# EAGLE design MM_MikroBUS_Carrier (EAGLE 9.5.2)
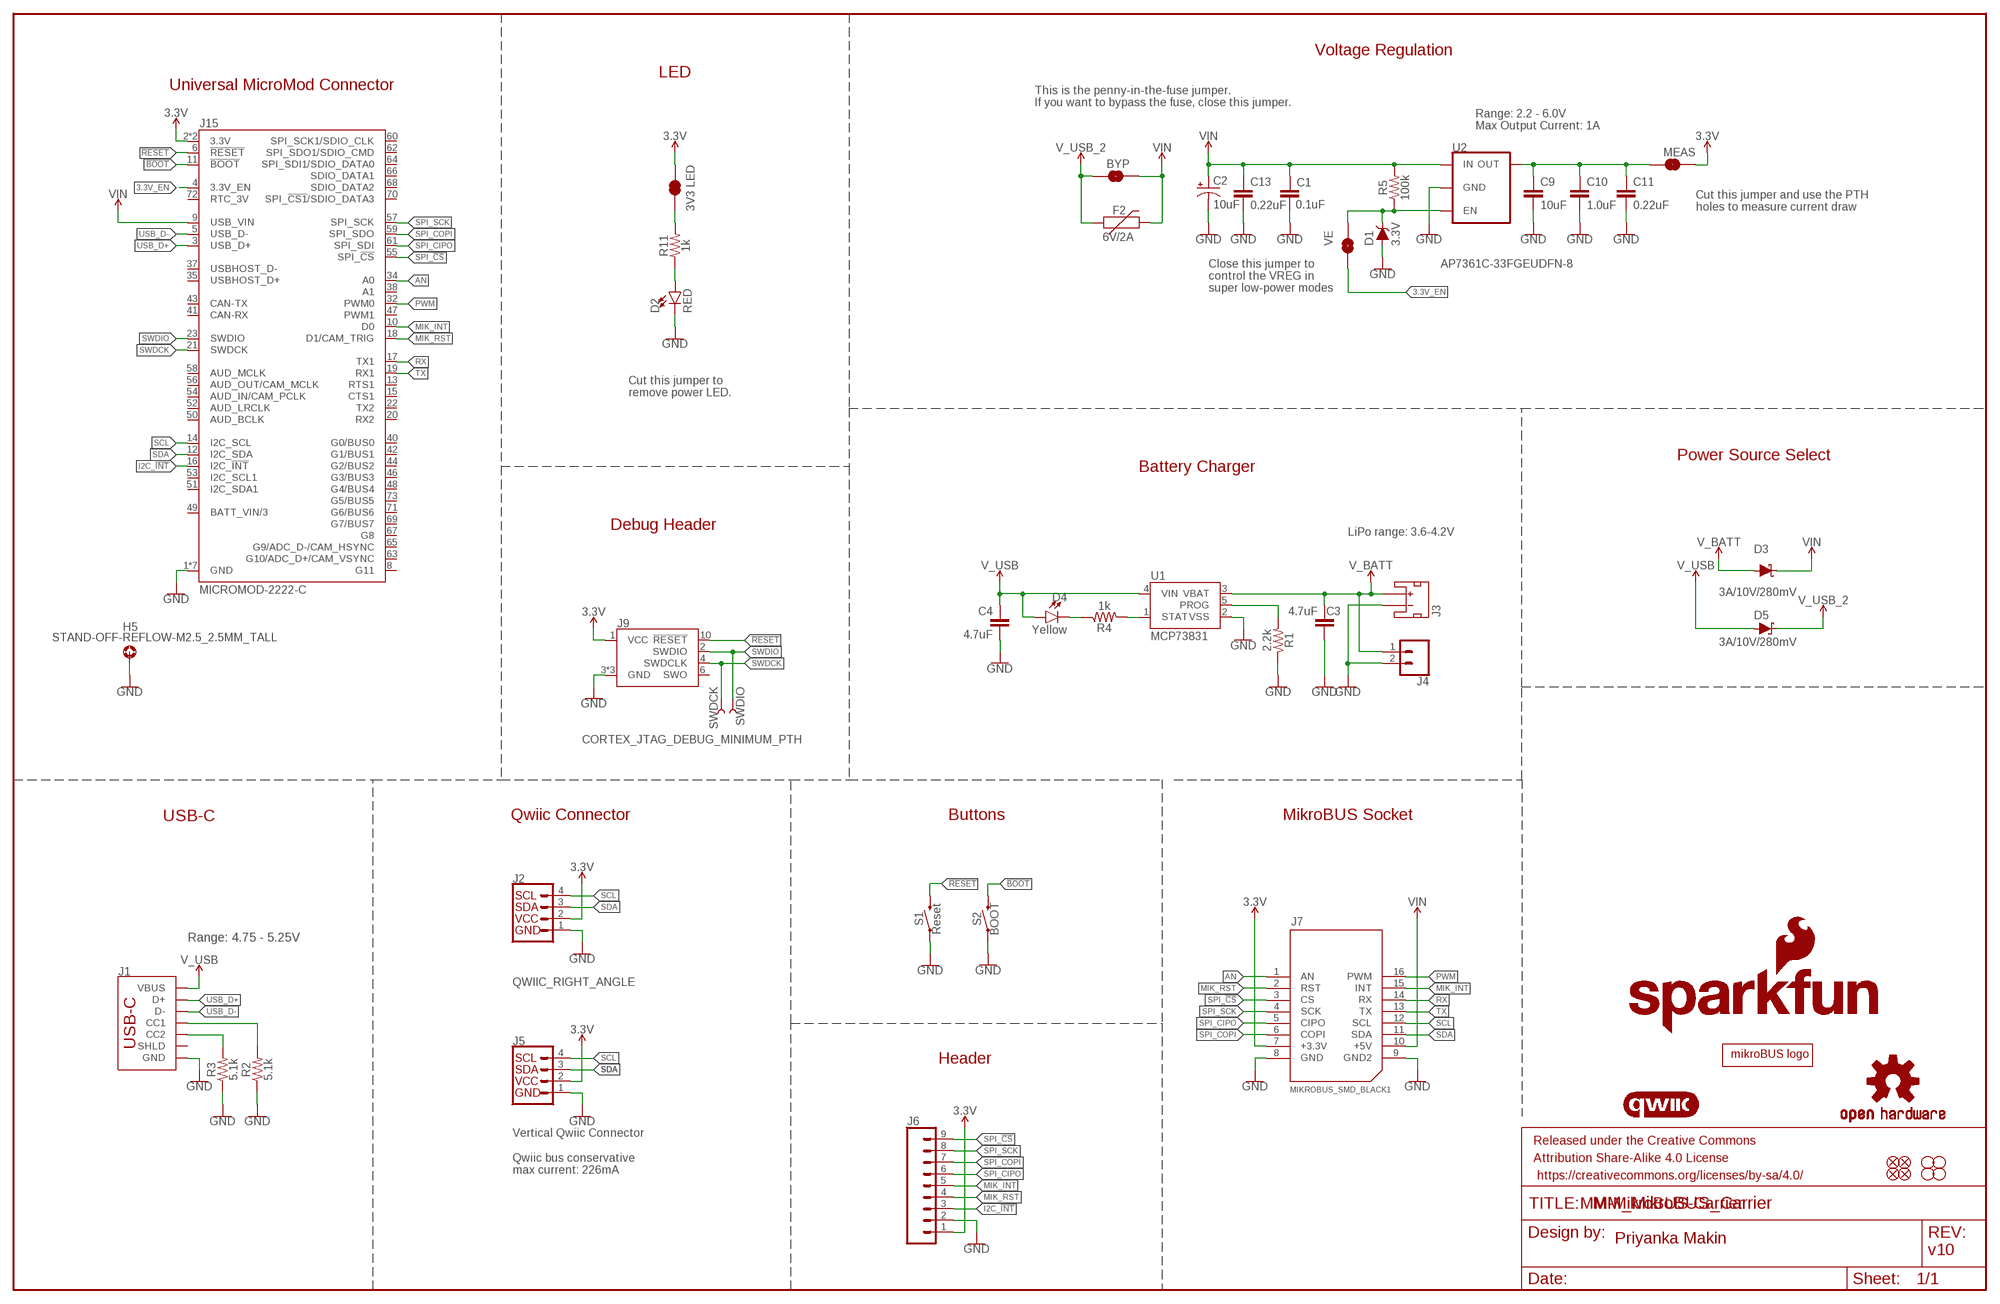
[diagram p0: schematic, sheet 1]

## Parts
BYP  JUMPER-SMT_2_NO_SILK  [SMT-JUMPER_2_NO_SILK]
C1  0.1uF  0.1UF-0603-25V-(+80/-20%)  [0603]
C2  10uF  10UF-POLAR-EIA3216-16V-10%(TANT)  [EIA3216]
C3  4.7uF  4.7UF-0603-35V-(20%)  [0603]
C4  4.7uF  4.7UF-0603-35V-(20%)  [0603]
C9  10uF  10UF-0603-6.3V-20%  [0603]
C10  1.0uF  1.0UF-0603-16V-10%  [0603]
C11  0.22uF  0.22UF-0603-25V-10%  [0603]
C13  0.22uF  0.22UF-0603-25V-10%  [0603]
D1  3.3V  DIODE-ZENER-MM3Z3V3T1G  [SOD-323]
D2  RED  LED-RED0603  [LED-0603]
D3  3A/10V/280mV  DIODE-SCHOTTKY-BAT60A  [SOD-323]
D4  Yellow  LED-YELLOW0603  [LED-0603]
D5  3A/10V/280mV  DIODE-SCHOTTKY-BAT60A  [SOD-323]
F2  6V/2A  PPTC_6V2A  [1210]
FD1  FIDUCIALUFIDUCIAL  [FIDUCIAL-MICRO]
FD2  FIDUCIALUFIDUCIAL  [FIDUCIAL-MICRO]
FD3  FIDUCIALUFIDUCIAL  [FIDUCIAL-MICRO]
FD4  FIDUCIALUFIDUCIAL  [FIDUCIAL-MICRO]
FRAME1  FRAME-LEDGER  [CREATIVE_COMMONS]
H1  STAND-OFF  [STAND-OFF]
H2  STAND-OFF  [STAND-OFF]
H3  STAND-OFF  [STAND-OFF]
H4  STAND-OFF  [STAND-OFF]
H5  STAND-OFF-REFLOW-M2.5_2.5MM_TALL  [STAND-OFF-REFLOW-M2.5]
J1  USB_C_2-LAYER_PADS  [USB-C-16P-2LAYER-PADS]
J2  QWIIC_RIGHT_ANGLE  QWIIC_CONNECTORJS-1MM  [JST04_1MM_RA]
J3  JST_2MM_MALE  [JST-2-SMD]
J4  CONN_021X02_NO_SILK  [1X02_NO_SILK]
J5  Vertical Qwiic Connector  QWIIC_CONNECTOR  [JST04_1MM_VERT]
J6  CONN_09NO_SILK  [1X09_NO_SILK]
J7  MIKROBUS_SMD_BLACK1  [MIKROBUS_SMD_BLACK]
J9  CORTEX_JTAG_DEBUG_MINIMUM_PTH  [2X5-PTH-1.27MM]
J15  MICROMOD-2222-C  [M.2-CONNECTOR-E]
JP4  3V3 LED  JUMPER-SMT_2_NC_TRACE_SILK  [SMT-JUMPER_2_NC_TRACE_SILK]
JP6  VE  JUMPER-SMT_2_NO_SILK  [SMT-JUMPER_2_NO_SILK]
LOGO1  SFE_LOGO_NAME_FLAME.2_INCH  [SFE_LOGO_NAME_FLAME_.2]
LOGO2  QWIIC_LOGO_CONNECTOR  [QWIIC_5.5MM]
LOGO3  OSHW-LOGOM  [OSHW-LOGO-M]
MEAS  JUMPER-COMBO_2_NC_TRACE  [COMBO-JUMPER_2_NC_TRACE]
R1  2.2k  2.2KOHM-0603-1/10W-1%  [0603]
R2  5.1k  5.1KOHM5.1KOHM-0603-1/10W-1%  [0603]
R3  5.1k  5.1KOHM5.1KOHM-0603-1/10W-1%  [0603]
R4  1k  1KOHM-0603-1/10W-1%  [0603]
R5  100k  100KOHM-0603-1/10W-1%  [0603]
R11  1k  1KOHM-0603-1/10W-1%  [0603]
S1  Reset  MOMENTARY-SWITCH-SPST-SMD-5.2-TALL-REDUNDANT  [TACTILE_SWITCH_SMD_5.2MM]
S2  BOOT  MOMENTARY-SWITCH-SPST-SMD-5.2-TALL-REDUNDANT  [TACTILE_SWITCH_SMD_5.2MM]
SWDCK  TEST-POINTTP_15TH_THRU  [TP_15TH]
SWDIO  TEST-POINTTP_15TH_THRU  [TP_15TH]
U1  MCP73831  [SOT23-5]
U2  AP7361C-33FGEUDFN-8  [UDFN-8]
U$7  MIKROBUS_LOGO  [MIKROBUS_LOGO]

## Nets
3.3V: J2.2 J5.2 J6.1 J7.7(+3.3V) J9.1(VCC) J15.2(3.3V) J15.74(3.3V) JP4.2 MEAS.2 MEAS.4
3.3V_EN: J15.4(3.3V_EN) JP6.1
!BOOT!: J15.11(!BOOT!) S2.3 S2.4
!RESET!: J9.10(!RESET) J15.6(!RESET!) S1.3 S1.4
AN: J7.1(AN) J15.34(A0)
GND: C1.2 C2.- C3.2 C4.2 C9.2 C10.2 C11.2 C13.2 D1.A D2.C H5.1 J1.GND J1.GND2(GND) J2.1 J3.1(-) J4.2 J5.1 J6.2 J7.8(GND) J7.9(GND2) J9.3(GND) J9.5(GND) J9.9(GND) J15.1(GND) J15.7(GND) J15.33(GND) J15.36(GND) J15.39(GND) J15.45(GND) J15.75(GND) R1.1 R2.1 R3.1 S1.1 S1.2 S2.1 S2.2 U1.2(VSS) U2.4(GND) U2.EP(GND)
I2C_!INT!: J6.3 J15.16(I2C_!INT!)
MIK_INT: J6.5 J7.15(INT) J15.10(D0)
MIK_RST: J6.4 J7.2(RST) J15.18(D1/CAM_TRIG)
N$1: C9.1 C10.1 C11.1 MEAS.1 MEAS.3 U2.1(OUT)
N$2: R1.2 U1.5(PROG)
N$3: D4.C R4.1
N$4: JP4.1 R11.2
N$6: D2.A R11.1
N$8: R4.2 U1.1(STAT)
N$10: J1.A5(CC1) R2.2
N$11: J1.B5(CC2) R3.2
PWM: J7.16(PWM) J15.32(PWM0)
RX: J7.14(RX) J15.17(TX1)
SCL: J2.4 J5.4 J7.12(SCL) J15.14(I2C_SCL)
SDA: J2.3 J5.3 J7.11(SDA) J15.12(I2C_SDA)
SPI_!CS!: J6.9 J7.3(CS) J15.55(SPI_!CS!)
SPI_CIPO: J6.6 J7.5(CIPO) J15.61(SPI_SDI)
SPI_COPI: J6.7 J7.6(COPI) J15.59(SPI_SDO)
SPI_SCK: J6.8 J7.4(SCK) J15.57(SPI_SCK)
SWDCK: J9.4(SWDCLK) J15.21(SWDCK) SWDCK.1
SWDIO: J9.2(SWDIO) J15.23(SWDIO) SWDIO.1
TX: J7.13(TX) J15.19(RX1)
USB_D+: J1.A6(D+) J1.B6(D+) J15.3(USB_D+)
USB_D-: J1.A7(D-) J1.B7(D-) J15.5(USB_D-)
V_BATT: C3.1 D3.A J3.2(+) J4.1 U1.3(VBAT)
V_USB: C4.1 D4.A D5.A J1.VBUS1(VBUS) J1.VBUS2(VBUS) U1.4(VIN)
V_USB_2: BYP.1 D5.C F2.1
VIN: BYP.2 C1.1 C2.+ C13.1 D3.C F2.2 J7.10(+5V) J15.9(USB_VIN) R5.2 U2.8(IN)
VREG_EN: D1.C JP6.2 R5.1 U2.5(EN)
Unconnected: J1.SHLD1(SHLD) J1.SHLD2(SHLD) J1.SHLD3(SHLD) J1.SHLD4(SHLD) J3.NC1(PAD1) J3.NC2(PAD2) J9.6(SWO) J15.8(G11) J15.13(RTS1) J15.15(CTS1) J15.20(RX2) J15.22(TX2) J15.35(USBHOST_D+) J15.37(USBHOST_D-) J15.38(A1) J15.40(G0/BUS0) J15.41(CAN-RX) J15.42(G1/BUS1) J15.43(CAN-TX) J15.44(G2/BUS2) J15.46(G3/BUS3) J15.47(PWM1) J15.48(G4/BUS4) J15.49(BATT_VIN/3) J15.50(AUD_BCLK) J15.51(I2C_SDA1) J15.52(AUD_LRCLK) J15.53(I2C_SCL1) J15.54(AUD_IN/CAM_PCLK) J15.56(AUD_OUT/CAM_MCLK) J15.58(AUD_MCLK) J15.60(SPI_SCK1/SDIO_CLK) J15.62(SPI_SDO1/SDIO_CMD) J15.63(G10/ADC_D+/CAM_VSYNC) J15.64(SPI_SDI1/SDIO_DATA0) J15.65(G9/ADC_D-/CAM_HSYNC) J15.66(SDIO_DATA1) J15.67(G8) J15.68(SDIO_DATA2) J15.69(G7/BUS7) J15.70(SPI_!CS1!/SDIO_DATA3) J15.71(G6/BUS6) J15.72(RTC_3V) J15.73(G5/BUS5)

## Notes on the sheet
- Voltage Regulation
- LED
- Universal MicroMod Connector
- This is the penny-in-the-fuse jumper.
  If you want to bypass the fuse, close this jumper.
- Range: 2.2 - 6.0V
  Max Output Current: 1A
- Cut this jumper and use the PTH 
  holes to measure current draw
- Close this jumper to 
  control the VREG in 
  super low-power modes
- Cut this jumper to
  remove power LED.
- Power Source Select
- Battery Charger
- Debug Header
- LiPo range: 3.6-4.2V
- USB-C | Qwiic Connector | Buttons | MikroBUS Socket
- Range: 4.75 - 5.25V
- Header
- Qwiic bus conservative 
  max current: 226mA
- MM-MikroBUS-Carrier
- Priyanka Makin
- v10

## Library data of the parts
BYP JP6 = SparkFun-Jumpers:JUMPER-SMT_2_NO: Normally open jumper
C1 = SparkFun-Capacitors:0.1UF: 0.1µF ceramic capacitors; PROD_ID: CAP-00810
C2 = SparkFun-Capacitors:10UF-POLAR: 10.0µF polarized capacitors; PROD_ID: CAP-00811
C3 C4 = SparkFun-Capacitors:4.7UF: 4.7µF ceramic capacitors; PROD_ID: CAP-14106
C9 = SparkFun-Capacitors:10UF: 10.0µF ceramic capacitors; PROD_ID: CAP-11015
C10 = SparkFun-Capacitors:1.0UF: 1µF ceramic capacitors; PROD_ID: CAP-00868
C11 C13 = SparkFun-Capacitors:0.22UF: 0.22µF ceramic capacitors; PROD_ID: CAP-07822
D1 = SparkFun-DiscreteSemi:DIODE-ZENER: Zener Diode; PROD_ID: DIO-11284
D2 = SparkFun-LED:LED-RED: Red SMD LED; PROD_ID: DIO-00819
D3 D5 = SparkFun-DiscreteSemi:DIODE-SCHOTTKY: Schottky diode; PROD_ID: DIO-14072
D4 = SparkFun-LED:LED-YELLOW: Yellow SMD LED; PROD_ID: DIO-09003
F2 = SparkFun-Fuses:PPTC: Resettable Fuse PPTC; PROD_ID: RES-14313
FD1-FD4 = SparkFun-Aesthetics:FIDUCIAL: Fiducial Alignment Points
FRAME1 = SparkFun-Aesthetics:FRAME-LEDGER: Schematic Frame - Ledger
H1-H4 = SparkFun-Hardware:STAND-OFF: Stand Off
H5 = SparkFun-Hardware:STAND-OFF-REFLOW: Stand Off Reflow Compatible; PROD_ID: HW-14899
J1 = SparkFun-Connectors:USB_C: USB Type C 16Pin Connector Super Speed pins not available on the 16-pin purely SMD connector so this part is best for USB 2.0 implementations. D1 and D2 are tied together enabling D+/- no matter which way the cable is plugged into the connector. The two channel configuration pins (CC1/2) are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; PROD_ID: CONN-14122
J2 = SparkFun-Connectors:QWIIC_CONNECTOR: SparkFun I2C Standard Qwiic Connector An SMD 1mm pitch JST connector makes it easy and quick (get it? Qwiic?) to connect I2C devices to each other. The Qwiic system enables fast and solderless connection between popular platforms and various sensors and actuators. We carry 200mm, 100mm, 50mm, and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; PROD_ID: CONN-13694
J3 = SparkFun-Connectors:JST_2MM_MALE: JST 2MM MALE RA CONNECTOR Two pin, compact surface mount connector. Commonly used as a battery input connection point. We really like the solid locking feeling and high current rating on these small connectors. We use these all the time as battery connectors. Mates to single-cell LiPo batteries.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; PROD_ID: CONN-11443; SF_ID: PRT-08612
J4 = SparkFun-Connectors:CONN_02: Multi connection point. Often used as Generic Header-pin footprint for 0.1 inch spaced/style header connections
J5 = SparkFun-Connectors:QWIIC_CONNECTOR: SparkFun I2C Standard Qwiic Connector An SMD 1mm pitch JST connector makes it easy and quick (get it? Qwiic?) to connect I2C devices to each other. The Qwiic system enables fast and solderless connection between popular platforms and various sensors and actuators. We carry 200mm, 100mm, 50mm, and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; PROD_ID: CONN-14483
J6 = SparkFun-Connectors:CONN_09: Multi connection point. Often used as Generic Header-pin footprint for 0.1 inch spaced/style header connections On any of the 0.1 inch spaced packages, you can populate with these: Break Away Headers - Straight (PRT-00116) Break Away Male Headers - Right Angle (PRT-00553) Female Headers (PRT-00115)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
J7 = mikroBUS_SMD_BLACK:MIKROBUS_SMD_BLACK; PROD_ID: CONN-16267
J9 = SparkFun-Connectors:CORTEX_JTAG_DEBUG_MINIMUM: Cortex Debug Connector - 10 pin Supports JTAG debug, Serial Wire debug, and Serial Wire Viewer. PTH and SMD connector options available. General Connector Information Products: PTH Connector -via Digi-Key SparkFun PSoc SparkFun T
J15 = SparkFun-MicroMod:MICROMOD: MicroMod Connector Description: A card edge connector and mating PCB connector to allow various MicroMod Processor Boards to be coupled with various carrier boards of different capabilities. Based on the M.2 standard.; PROD_ID: CONN-14877
JP4 = SparkFun-Jumpers:JUMPER-SMT_2_NC_TRACE: Normally closed trace jumper
LOGO1 = SparkFun-Aesthetics:SFE_LOGO_NAME_FLAME: SparkFun Font Logo w/ Flame
LOGO2 = SparkFun-Aesthetics:QWIIC_LOGO: Qwiic Logos for placement on schematic and PCB. The 5.5mm silk logo is best for placing next to Qwiic connector.
LOGO3 = SparkFun-Aesthetics:OSHW-LOGO: Open-Source Hardware (OSHW) Logo
MEAS = SparkFun-Jumpers:JUMPER-COMBO_2_NC_TRACE
R1 = SparkFun-Resistors:2.2KOHM: 2.2kΩ resistor; PROD_ID: RES-08272
R2 R3 = SparkFun-Resistors:5.1KOHM; PROD_ID: RES-12083
R4 R11 = SparkFun-Resistors:1KOHM: 1kΩ resistor; PROD_ID: RES-07856
R5 = SparkFun-Resistors:100KOHM: 100kΩ resistor; PROD_ID: RES-07828
S1 S2 = SparkFun-Switches:MOMENTARY-SWITCH-SPST: Momentary Switch (Pushbutton) - SPST; PROD_ID: SWCH-14139
SWDCK SWDIO = SparkFun-Connectors:TEST-POINT: SparkFun Test Points
U1 = SparkFun-IC-Power:MCP73831: MCP73831T Li-Ion, Li-Pol Controller Miniature single cell, fully integrated Li-Ion, Li-polymer charge management controller Datasheet SparkFun Products: SparkFun ESP32 Thing SparkFun 9DoF Razor IMU M0; PROD_ID: IC-09995
U2 = SparkFun-IC-Power:AP7361C-33FGE: AP7361C 3.3V LDO Regulator; PROD_ID: VREG-14094
U$7 = mikroBUS_SMD_BLACK:MIKROBUS_LOGO

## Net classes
0 default: width 0 mm, drill 0 mm
1 power: width 0.762 mm

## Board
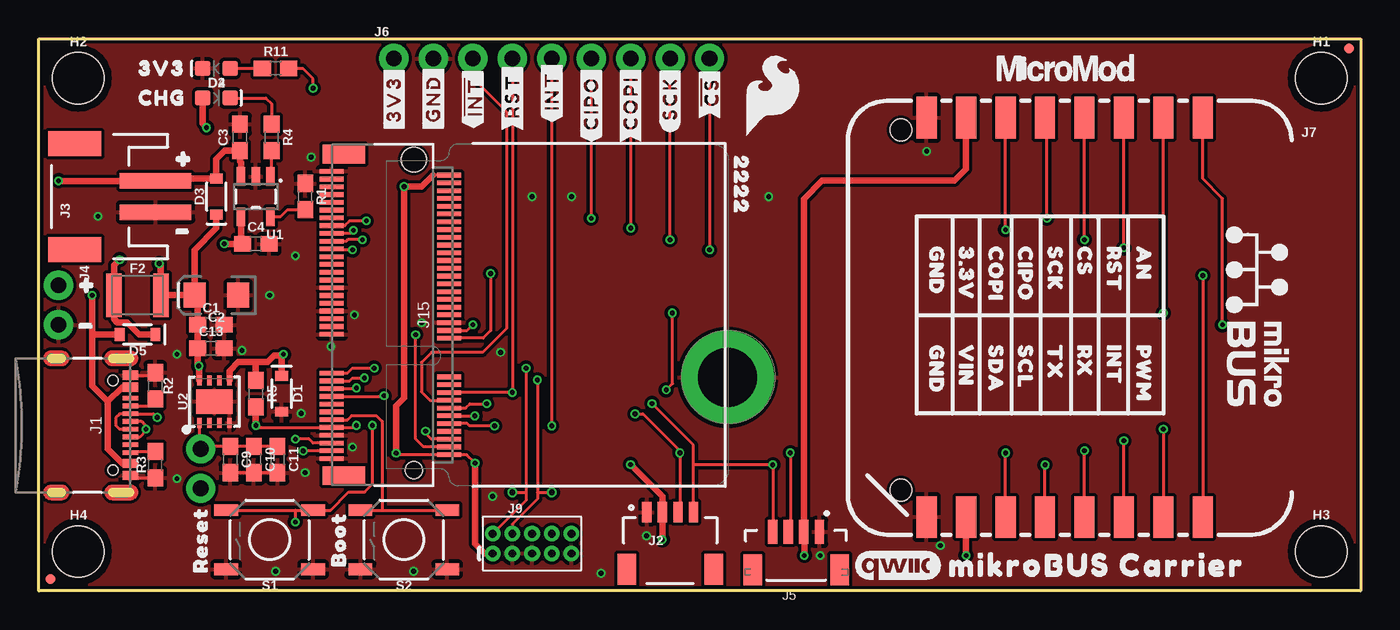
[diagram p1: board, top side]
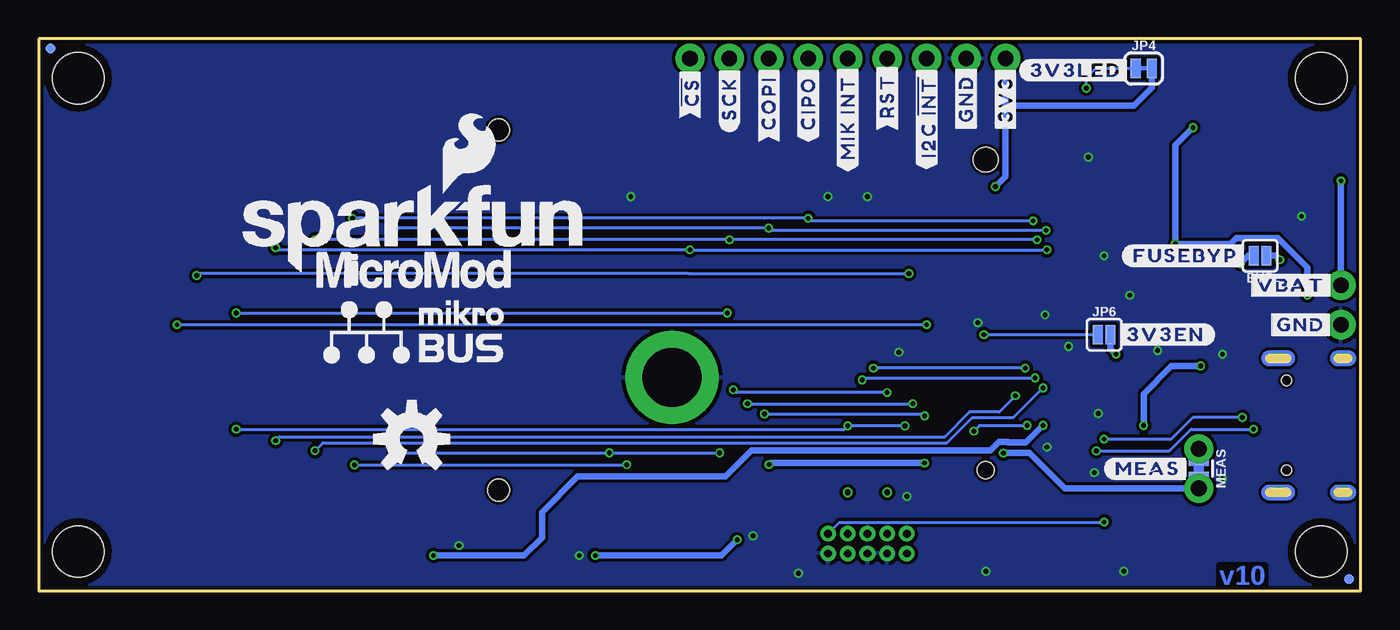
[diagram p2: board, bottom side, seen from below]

Size 85.09 x 35.56 mm. Coordinates in mm from the lower left corner, seen from the top.
Outline: 0,0 0,35.56 85.09,35.56 85.09,0 0,0
Copper layers (1*16): Top 0.035mm / dielectric 1.5mm / Bottom 0.035mm
Design rules "SparkFun-2-Layer-Minimum-JLCPCB": minimum track width 5mil, minimum drill 0.3mm, track to track 5mil, track to pad 5mil, pad to pad 5mil, via to via 5mil, smd to smd 5mil, copper to edge 7mil, drill to drill 7mil, minimum pad ring 5mil, minimum via ring 5mil, stop-mask expansion 2.5mil, vias tented up to drill 25mil, thermal gap 10mil

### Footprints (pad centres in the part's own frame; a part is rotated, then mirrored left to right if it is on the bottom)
SMT-JUMPER_2_NO_SILK = smd 0.635 x 1.27: 1 -0.406,0; 2 0.406,0
0603 = smd 1.1 x 1: 1 -0.85,0; 2 0.85,0
EIA3216 = smd 1.4 x 1.6: + 1.4,0; - -1.4,0
SOD-323 = smd 0.63 x 0.83: A 1.15,0; C -1.15,0
LED-0603 = smd 1 x 1: A -0.877,0; C 0.877,0
1210 = smd 1 x 2.8: 1 -1.5,0; 2 1.5,0
FIDUCIAL-MICRO = smd 0.635 x 0.635: 1 0,0
STAND-OFF = hole 3.302: 0,0
STAND-OFF-REFLOW-M2.5 = drill 3.8 pad 6: 1 0,0
USB-C-16P-2LAYER-PADS = smd 0.3 x 1: A5 -1.25,-0.34; A6 -0.25,-0.34; A7 0.25,-0.34; A8 1.25,-0.34; B5 1.75,-0.34; B6 0.75,-0.34; B7 -0.75,-0.34; B8 -1.75,-0.34 | smd 0.6 x 1: GND -3.225,-0.34; GND2 3.225,-0.34; VBUS1 -2.45,-0.34; VBUS2 2.45,-0.34 | drill 0.4 pad 0.6 long: SHLD1 -4.318,-0.915; SHLD2 4.318,-0.915; SHLD3 -4.318,-5.095; SHLD4 4.318,-5.095 | hole 0.65: -2.89,-1.445; 2.89,-1.445
JST04_1MM_RA = smd 0.6 x 1.35: 1 -1.5,0; 2 -0.5,0; 3 0.5,0; 4 1.5,0 | smd 1.2 x 2: NC1 2.8,-3.675; NC2 -2.8,-3.675
JST-2-SMD = smd 1 x 4.6: 1 -1,-3.7; 2 1,-3.7 | smd 1.6 x 3.4: NC1 -3.4,1.5; NC2 3.4,1.5
1X02_NO_SILK = drill 1.016 pad 1.88: 1 0,0; 2 2.54,0
JST04_1MM_VERT = smd 0.6 x 1.55: 1 -1.478,0.775; 2 -0.478,0.775; 3 0.522,0.775; 4 1.522,0.775 | smd 1.2 x 2: NC1 -2.778,3.2; NC2 2.822,3.2
1X09_NO_SILK = drill 1.016 pad 1.88: 1 0,0; 2 2.54,0; 3 5.08,0; 4 7.62,0; 5 10.16,0; 6 12.7,0; 7 15.24,0; 8 17.78,0; 9 20.32,0
MIKROBUS_SMD_BLACK = smd 2.7 x 1.3: 1 -12.7,8.89; 2 -12.7,6.35; 3 -12.7,3.81; 4 -12.7,1.27; 5 -12.7,-1.27; 6 -12.7,-3.81; 7 -12.7,-6.35; 8 -12.7,-8.89; 9 13.02,-8.89; 10 13.02,-6.35; 11 13.02,-3.81; 12 13.02,-1.27; 13 13.02,1.27; 14 13.02,3.81; 15 13.02,6.35; 16 13.02,8.89 | hole 1.4: -11.914,-10.541; 11.286,-10.541
2X5-PTH-1.27MM = drill 0.508 pad 1: 1 -2.54,-0.635; 2 -2.54,0.635; 3 -1.27,-0.635; 4 -1.27,0.635; 5 0,-0.635; 6 0,0.635; 7 1.27,-0.635; 8 1.27,0.635; 9 2.54,-0.635; 10 2.54,0.635
M.2-CONNECTOR-E = smd 0.3 x 1.55: 1 9.25,-5.275; 2 9,2.275; 3 8.75,-5.275; 4 8.5,2.275; 5 8.25,-5.275; 6 8,2.275; 7 7.75,-5.275; 8 7.5,2.275; 9 7.25,-5.275; 10 7,2.275; 11 6.75,-5.275; 12 6.5,2.275; 13 6.25,-5.275; 14 6,2.275; 15 5.75,-5.275; 16 5.5,2.275; 17 5.25,-5.275; 18 5,2.275; 19 4.75,-5.275; 20 4.5,2.275; 21 4.25,-5.275; 22 4,2.275; 23 3.75,-5.275; 32 1.5,2.275; 33 1.25,-5.275; 34 1,2.275; 35 0.75,-5.275; 36 0.5,2.275; 37 0.25,-5.275; 38 0,2.275; 39 -0.25,-5.275; 40 -0.5,2.275; 41 -0.75,-5.275; 42 -1,2.275; 43 -1.25,-5.275; 44 -1.5,2.275; 45 -1.75,-5.275; 46 -2,2.275; 47 -2.25,-5.275; 48 -2.5,2.275; 49 -2.75,-5.275; 50 -3,2.275; 51 -3.25,-5.275; 52 -3.5,2.275; 53 -3.75,-5.275; 54 -4,2.275; 55 -4.25,-5.275; 56 -4.5,2.275; 57 -4.75,-5.275; 58 -5,2.275; 59 -5.25,-5.275; 60 -5.5,2.275; 61 -5.75,-5.275; 62 -6,2.275; 63 -6.25,-5.275; 64 -6.5,2.275; 65 -6.75,-5.275; 66 -7,2.275; 67 -7.25,-5.275; 68 -7.5,2.275; 69 -7.75,-5.275; 70 -8,2.275; 71 -8.25,-5.275; 72 -8.5,2.275; 73 -8.75,-5.275; 74 -9,2.275; 75 -9.25,-5.275 | smd 1.2 x 2.75: A1 10.35,-4.5; A2 -10.35,-4.5 | hole 1.1: 10,0 | hole 1.6: -10,0
SMT-JUMPER_2_NC_TRACE_SILK = smd 0.66 x 1.27: 1 -0.521,0; 2 0.521,0
COMBO-JUMPER_2_NC_TRACE = smd 0.635 x 1.27: 1 -0.508,0; 2 0.508,0 | drill 1.016 pad 1.88: 3 -1.27,0; 4 1.27,0
TACTILE_SWITCH_SMD_5.2MM = smd 1.524 x 0.762: 1 -2.794,1.905; 2 2.794,1.905; 3 -2.794,-1.905; 4 2.794,-1.905
TP_15TH = drill 0.381 pad 0.61: 1 0,0
SOT23-5 = smd 0.55 x 1.2: 1 -0.95,-1.3; 2 0,-1.3; 3 0.95,-1.3; 4 0.95,1.3; 5 -0.95,1.3
UDFN-8 = smd 0.3 x 0.65: 1 -0.975,-1.375; 2 -0.325,-1.375; 3 0.325,-1.375; 4 0.975,-1.375; 5 0.975,1.375; 6 0.325,1.375; 7 -0.325,1.375; 8 -0.975,1.375 | smd 2.35 x 1.6: EP 0,0

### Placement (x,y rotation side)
BYP  6.48,21.59 180 bottom
C1  11.09,17.14 0 top
C2  11.43,19.05 180 top
C3  12.95,29.21 90 top
C4  13.97,22.35 0 top
C9  12.32,8.47 270 top
C10  13.84,8.47 270 top
C11  15.37,8.47 270 top
C13  11.09,15.62 0 top
D1  15.62,12.7 270 top
D2  11.43,33.66 180 top
D3  11.43,25.4 90 top
D4  11.43,31.75 0 top
D5  6.35,16.51 180 top
F2  6.35,19.05 0 top
FD1  0.76,0.76 0 top
FD2  84.33,34.92 0 top
FD3  0.76,0.76 0 bottom
FD4  84.33,34.92 0 bottom
FRAME1  not placed on the board
H1  82.55,33.02 0 top
H2  2.54,33.02 0 top
H3  82.55,2.54 0 top
H4  2.54,2.54 0 top
H5  44.33,13.76 0 top
J1  6.22,10.67 270 top
J2  40.64,5.08 0 top
J3  3.81,25.4 90 top
J4  1.27,19.68 270 top
J5  48.77,4.57 180 top
J6  22.86,34.29 0 top
J7  66.04,17.78 270 top
J9  31.75,3.05 0 top
J15  24.13,17.78 270 top
JP4  13.97,33.66 0 bottom
JP6  16.51,16.51 0 bottom
LOGO1  60.96,23.37 0 bottom
LOGO2  55.31,1.65 0 top
LOGO3  61.09,9.78 0 bottom
MEAS  10.41,7.87 270 bottom
R1  17.14,25.4 270 top
R2  7.49,13.21 270 top
R3  7.49,8.13 90 top
R4  14.99,29.21 270 top
R5  13.97,12.7 270 top
R11  15.24,33.66 0 top
S1  14.86,3.3 180 top
S2  23.5,3.3 180 top
SWDCK  33.02,6.35 0 top
SWDIO  30.48,6.35 0 top
U1  13.97,25.4 180 top
U2  11.3,12.19 0 top
U$1  [#3V3LED#0]  21.97,33.53 0 bottom
U$2  [MICROMOD_LOGO_.35]  66.04,33.66 0 top
U$3  [3V30]  5.71,33.66 0 top
U$4  [CHG0]  5.71,31.75 0 top
U$5  [MIKROBUS_CARRIER0]  57.53,1.65 0 top
U$6  [#INT#0]  33.02,30.23 90 top
U$7  61.09,17.02 0 bottom
U$8  [#GND#0]  25.4,29.46 90 top
U$9  [#MEAS#0]  16.51,7.87 0 bottom
U$10  [#3V3#0]  22.86,29.46 90 top
U$11  [#0]  1.52,19.68 0 top
U$12  [#VBAT#0]  7.37,19.68 0 bottom
U$13  [#3V3#0]  22.86,29.46 90 bottom
U$14  [#GND#0]  25.4,29.46 90 bottom
U$15  [##INT##0]  27.94,29.84 90 top
U$16  [#MIK_INT#0]  33.02,27.05 90 bottom
U$17  [#RST#0]  30.48,29.72 90 top
U$18  [#RST#0]  30.48,29.72 90 bottom
U$20  [#I2C_#INT##0]  27.94,27.18 90 bottom
U$22  [#CIPO#0]  35.56,28.96 90 top
U$23  [#CIPO#0]  35.56,28.96 90 bottom
U$24  [#COPI#0]  38.1,28.96 90 top
U$25  [#COPI#0]  38.1,28.96 90 bottom
U$26  [#SCK#0]  40.64,29.59 90 top
U$27  [#SCK#0]  40.64,29.59 90 bottom
U$28  [##CS##0]  43.18,30.48 90 top
U$29  [##CS##0]  43.18,30.48 90 bottom
U$30  [RESET0]  10.41,0.51 90 top
U$31  [BOOT0]  19.3,0.89 90 top
U$32  [#0]  7.75,27.81 0 top
U$33  [#GND#0]  6.1,17.14 0 bottom
U$34  [22220]  45.21,28.7 270 top
U$35  [AN0]  71.12,22.86 270 top
U$36  [#0]  1.14,17.4 0 top
U$37  [#0]  7.37,23.5 0 top
U$38  [#FUSEBYP#0]  15.37,21.59 0 bottom
U$39  [#3V3EN#0]  15.75,16.51 0 bottom
U$40  [RST0]  69.22,22.86 270 top
U$41  [CS0]  67.31,22.86 270 top
U$42  [SCK0]  65.41,22.86 270 top
U$43  [CIPO0]  63.5,22.86 270 top
U$44  [SFE_LOGO_FLAME_.2]  47.24,31.88 0 top
U$45  [COPI0]  61.59,22.86 270 top
U$46  [3#3V0]  59.69,22.86 270 top
U$47  [GND0]  57.78,22.86 270 top
U$48  [GND0]  57.78,16.51 270 top
U$49  [PWM0]  71.12,16.51 270 top
U$50  [INT0]  69.22,16.51 270 top
U$51  [RX0]  67.31,16.51 270 top
U$52  [TX0]  65.41,16.51 270 top
U$53  [SCL0]  63.5,16.51 270 top
U$54  [SDA0]  61.59,16.51 270 top
U$55  [VIN0]  59.69,16.51 270 top
U$68  [MICROMOD_LOGO_.5]  60.96,20.7 0 bottom

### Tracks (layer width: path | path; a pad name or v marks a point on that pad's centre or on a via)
3.3V  (via drill 0.3)
  Top 0.203: v23,8.88 23.1,8.78 J15.2 27.54,8.78 v28.08,8.24 | J15.74 25.38,26.78
  Top 0.406: v38.08,8.14 40.14,6.09 J2.2 v40.14,3.31 v40.13,3.3 | v23,8.88 23,11.93 23.51,12.43 v23.51,26.05 24.65,26.05 25.38,26.78 | v49.28,2.29 49.28,3.77 J5.2 49.25,25.24 50.42,26.42 58.93,26.42 59.69,27.18 J7.7 | v28.08,8.24 28.08,3.04 28.7,2.41 J9.1
  Bottom 0.203: MEAS.2 MEAS.4 | v23,8.88 22.99,8.89
  Bottom 0.406: MEAS.4 19.05,6.6 21.34,8.89 22.99,8.89 | JP4.2 13.45,32.4 14.61,31.24 22.86,31.24 | v40.13,3.3 41.15,2.29 v49.28,2.29 | J6.1 22.86,31.24 | 22.86,31.24 22.86,26.7 v23.51,26.05 | v38.08,8.14 37.99,8.24 v28.08,8.24
3.3V_EN  (via drill 0.3)
  Top 0.203: J15.4 24.76,9.28 24.26,9.78 v24.26,16.51
  Bottom 0.203: v24.26,16.51 JP6.1
!BOOT!
  Top 0.203: S2.4 22.1,5.21 | 22.1,5.21 S2.3 | J15.11 19.87,11.03 20.12,11.28 21.74,11.28 22.1,10.92 22.1,5.21
!RESET!  (via drill 0.3)
  Top 0.203: v24.89,10.29 24.89,10.15 25.26,9.78 J15.6 | v21.46,10.67 21.46,6.86 20.98,6.38 19.95,6.38 18.78,5.21 S1.3 16.51,5.21 | S1.4 16.51,5.21 | 16.51,5.21 v16.51,4.45
  Bottom 0.203: v24.89,10.29 24.51,10.67 v21.46,10.67 | v16.51,4.45 16.54,4.41 33.56,4.41 J9.10
AN  (via drill 0.3)
  Top 0.203: J15.34 27.57,16.78 v27.94,17.14 | v76.2,17.14 76.2,25.27 74.93,26.54 J7.1
  Bottom 0.203: v27.94,17.14 v76.2,17.14
GND  (via drill 0.3)
  Top 0.203: J1.GND 7.33,13.89 R2.1 | J1.GND2 6.05,7.28 R3.1 | C9.2 C10.2 C11.2
  other vias: 17.53,27.94 3.81,24.13 16.51,21.59 14.86,19.05 8.89,15.24 8.89,7.24 15.24,1.27 17.14,7.62 20.19,9.27 39.12,3.56 18.8,15.75 24.64,17.27 57.15,28.32 58.04,2.92 36.2,1.14 50.29,2.29 24.13,1.27 13.08,15.49 16.89,11.43 20.32,17.78 34.29,25.4 46.99,25.4 31.75,25.4 29.72,15.37 29.21,6.1
  pour Top (isolate 0.203): 0,35.56 0,0 85.09,0 85.09,35.56
  pour Bottom (isolate 0.203): 0,35.56 0,0 85.09,0 85.09,35.56
I2C_!INT!
  Top 0.203: J15.16 25.18,12.28 24.64,12.83 24.64,14.73 25.27,15.37 28.57,15.37 30.1,16.89 30.1,30.86 27.94,33.02 J6.3
MIK_INT  (via drill 0.3)
  Top 0.203: v29.34,10.63 27.72,10.63 27.57,10.78 J15.10 | v72.39,10.41 J7.15 | J6.5 v33.02,10.63
  Bottom 0.203: v29.34,10.63 29.65,10.63 29.68,10.67 33.02,10.67 v33.02,10.63 33.24,10.41 v72.39,10.41
MIK_RST  (via drill 0.3)
  Top 0.203: J15.18 v30.48,12.78 J6.4 | v40.39,12.95 40.79,13.36 40.79,17.88 v40.77,17.91 | v72.39,17.91 J7.2
  Bottom 0.203: v72.39,17.91 v40.77,17.91 | v30.48,12.78 40.21,12.78 v40.39,12.95
N$1
  Top 0.203: C11.1 C10.1 C9.1 11.3,9.32 11.13,9.14 MEAS.3 10.33,9.23 U2.1
  Bottom 0.203: MEAS.1 MEAS.3
N$2
  Top 0.203: U1.5 15.55,24.1 16,24.55 R1.2
N$3
  Top 0.203: D4.C 14.61,31.75 14.99,31.37 R4.1
N$4  (via drill 0.3)
  Top 0.203: v17.65,32.38 17.65,32.98 16.98,33.66 R11.2
  Bottom 0.203: v17.65,32.38 17.65,33.03 17.03,33.66 JP4.1
N$6
  Top 0.203: D2.A R11.1
N$8
  Top 0.203: U1.1 14.99,26.77 R4.2
N$10
  Top 0.203: J1.A5 7.05,11.92 R2.2
N$11
  Top 0.203: J1.B5 5.94,8.98 R3.2
PWM  (via drill 0.3)
  Top 0.203: v29.08,20.45 29.08,16.76 28.6,16.28 J15.32 | v74.93,20.32 J7.16
  Bottom 0.203: v29.08,20.45 43.18,20.45 43.31,20.45 74.8,20.45 v74.93,20.32
RX  (via drill 0.3)
  Top 0.203: J15.17 22.18,12.53 v22.23,12.57 | J7.14 v69.85,9.68
  Bottom 0.203: v22.23,12.57 23.27,11.53 25.18,11.53 26.78,9.93 69.6,9.93 v69.85,9.68
SCL  (via drill 0.3)
  Top 0.203: J2.4 42.14,8.13 | 42.14,8.13 42.14,9.4 v39.47,12.06 | 42.14,8.13 v47.25,8.13 J5.4 | J7.12 v64.77,8.12 | J15.14 27.48,11.78 27.75,12.05 v28.83,12.05
  Bottom 0.203: v47.25,8.13 47.26,8.11 v64.77,8.11 v64.77,8.12 | v28.83,12.05 39.34,12.05 39.35,12.06 v39.47,12.06
SDA  (via drill 0.3)
  Top 0.203: J2.3 41.27,5.21 v41.27,8.89 41.27,9.03 38.88,11.41 v38.38,11.41 | v48.37,8.89 48.37,3.92 J5.3 | J7.11 v62.23,8.89 | J15.12 v28.07,11.28
  Bottom 0.203: v62.23,8.89 v48.37,8.89 v41.27,8.89 | v28.07,11.28 28.19,11.41 v38.38,11.41
SPI_!CS!  (via drill 0.3)
  Top 0.203: v20.19,21.97 18.91,21.97 J15.55 | v69.85,22.1 J7.3 | J6.9 v43.18,21.97
  Bottom 0.203: v20.19,21.97 v43.18,21.97 69.72,21.97 v69.85,22.1
SPI_CIPO  (via drill 0.3)
  Top 0.203: J15.61 19.69,23.53 20,23.84 v21.08,23.84 | J6.6 v35.56,24 | J7.5 64.9,30.35 v64.9,24
  Bottom 0.203: v21.08,23.84 35.56,23.84 v35.56,24 37.82,24 37.83,24.02 38.37,24.02 38.38,24 v64.9,24
SPI_COPI  (via drill 0.3)
  Top 0.203: v20.25,23.23 20.05,23.03 J15.59 | J6.7 v38.1,23.37 | v62.23,23.27 J7.6
  Bottom 0.203: v20.25,23.23 38.1,23.23 v38.1,23.37 62.13,23.37 v62.23,23.27
SPI_SCK  (via drill 0.3)
  Top 0.203: v20.83,22.62 19.89,22.62 19.8,22.53 J15.57 | v67.31,22.62 J7.4 | v40.63,22.62 40.63,34.28 J6.8
  Bottom 0.203: v20.83,22.62 v40.63,22.62 v67.31,22.62
SWDCK  (via drill 0.3)
  Top 0.203: J15.21 20.01,13.53 20.19,13.72 v20.95,13.72 | v32.09,13.59 32.09,6.35 | 32.09,6.35 32.09,5.93 30.48,4.32 J9.4 | 32.09,6.35 SWDCK.1
  Bottom 0.203: v20.95,13.72 32.22,13.72 v32.09,13.59
SWDIO  (via drill 0.3)
  Top 0.203: J15.23 19.87,14.03 20.19,14.35 v21.59,14.35 | v31.37,14.35 31.37,6.35 | 31.37,6.35 31.37,5.84 J9.2 | SWDIO.1 31.37,6.35
  Bottom 0.203: v21.59,14.35 v31.37,14.35
TX  (via drill 0.3)
  Top 0.203: J15.19 20.4,13.03 v20.45,13.08 | J7.13 v67.31,9.03
  Bottom 0.203: v20.45,13.08 22.38,11.15 25.02,11.15 26.63,9.54 66.8,9.54 v67.31,9.03
USB_D+  (via drill 0.3)
  Top 0.203: J1.A6 6.61,10.92 6.86,10.67 6.86,10.45 v6.89,10.41 6.89,10.32 6.48,9.91 5.89,9.91 J1.B6 | J15.3 v17.03,9.03 v17.02,9.02
  Bottom 0.203: v17.02,9.02 12.32,9.02 10.92,10.41 v6.89,10.41
USB_D-  (via drill 0.3)
  Top 0.203: J1.A7 5.2,10.42 4.95,10.67 4.95,11.18 5.2,11.42 J1.B7 7.38,11.42 v7.62,11.17 | J15.5 17.65,9.53 17.4,9.78 v16.51,9.78
  Bottom 0.203: v7.62,11.17 10.79,11.17 12.19,9.78 v16.51,9.78
V_BATT  (via drill 0.3)
  Top 0.406: U1.3 13.02,27.59 12.95,27.66 C3.1 11.98,28.36 11.43,27.81 D3.A 7.66,26.55 J3.2 1.29,26.4 v1.27,26.42
  Bottom 0.406: v1.27,26.42 J4.1
V_USB  (via drill 0.3)
  Top 0.406: J1.VBUS2 5.37,8.22 4.45,9.14 4.45,12.19 | J1.VBUS1 5.37,13.12 4.45,12.19 | 4.45,12.19 3.43,13.21 3.43,16.51 | v3.43,19.05 3.43,16.51 | v11.94,22.35 C4.1 13.02,22.45 U1.4 | D4.A 10.55,30.09 v10.79,29.84 | D5.A 3.43,16.51
  Bottom 0.406: v3.43,19.05 3.43,20.83 5.33,22.73 8,22.73 8.38,22.35 v11.94,22.35 11.94,28.7 v10.79,29.84
V_USB_2  (via drill 0.3)
  Top 0.406: D5.C 6.47,16.51 5.67,17.31 5.05,17.31 4.85,17.5 F2.1 4.85,20.98 v5.21,21.34
  Bottom 0.406: v5.21,21.34 5.46,21.59 BYP.1
VIN  (via drill 0.3)
  Top 0.203: v13.97,10.67 13.97,10.66 14.1,10.53 J15.9 20.31,10.53 v20.45,10.67
  Top 0.406: C2.+ F2.2 7.85,20.98 v7.75,21.08 | C2.+ 10.24,18.84 C1.1 C13.1 10.24,14.55 v10.3,14.49 10.33,14.46 U2.8 | R5.2 v13.97,10.67 | D3.C 11.43,23.37 10.03,21.97 C2.+ | v59.69,2.29 J7.10
  Bottom 0.406: v7.75,21.08 7.24,21.59 BYP.2 | v10.3,14.49 12.18,14.49 13.97,12.7 v13.97,10.67 | v20.45,10.67 21.54,9.58 22.69,9.58 22.71,9.59 23.3,9.59 23.83,9.05 39.2,9.05 40.89,7.37 50.42,7.37 52.7,5.08 52.7,3.43 53.85,2.29 v59.69,2.29
VREG_EN  (via drill 0.3)
  Top 0.406: D1.C 15.62,15.11 15.68,15.18 | 15.68,15.18 v15.75,15.24 | R5.1 13.97,14.73 13.96,14.74 | U2.5 12.28,14.18 12.84,14.74 13.96,14.74 | 13.96,14.74 14.72,14.74 15.16,15.18 15.68,15.18
  Bottom 0.406: v15.75,15.24 16.1,15.6 JP6.2

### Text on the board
Bottom: v10
Measures: All units in inches.
tDocu: Priyanka Makin

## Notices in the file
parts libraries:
SparkFun-Aesthetics: Licensing: Creative Commons ShareAlike 4.0 International - https://creativecommons.org/licenses/by-sa/4.0
SparkFun-Aesthetics: Released under the Creative Commons Attribution Share-Alike 4.0 License
SparkFun-Aesthetics: https://creativecommons.org/licenses/by-sa/4.0
